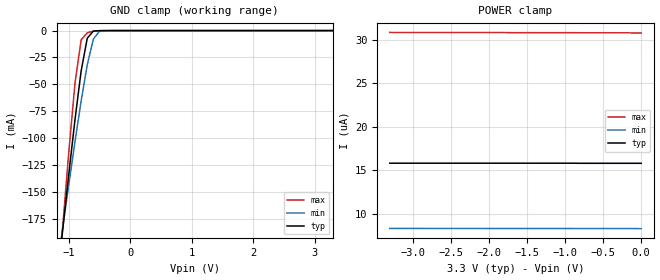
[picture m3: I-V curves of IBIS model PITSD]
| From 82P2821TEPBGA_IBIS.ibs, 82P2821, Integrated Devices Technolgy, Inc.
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|   Model PITSD
[Model]		PITSD
Model_type	Input
Polarity   Non-Inverting
Vinl = 		0.8000V
Vinh = 		2.0000V
C_comp   4.8700pF   4.3000pF   5.3800pF
[Temperature Range]	  25.0000   90.0000   -40.0000
[Voltage Range]   3.3000V   3.0000V   3.6000V
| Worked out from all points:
|   GND clamp passes 1 mA (typ) near -0.61 V on its own axis
[GND_clamp]
|Voltage	  I(typ)   I(min)   I(max)
-3.3V     -1.417A    -1.129A    -1.858A
-1.2V     -239.2mA   -225mA     -255.1mA
-1.1V     -185.7mA   -183.7mA   -182.6mA
-1V       -133.3mA   -143.1mA   -112.7mA
-900mV    -83.07mA   -103.5mA   -49.11mA
-800mV    -37.76mA   -65.72mA   -8.683mA
-700mV    -7.08mA    -31.79mA   -2.043mA
-600mV    -441.5uA   -7.708mA   -455.2uA
-500mV    -36.4uA    -560.8uA   -62.09uA
3.3V      15.8uA     8.301uA    30.77uA
[POWER_clamp]
|Voltage	  I(typ)   I(min)   I(max)
-3.3V     15.81uA    8.312uA    30.84uA
-3.2V     15.81uA    8.312uA    30.83uA
-2.6V     15.81uA    8.309uA    30.83uA
-2.5V     15.81uA    8.309uA    30.82uA
-1.8V     15.81uA    8.307uA    30.82uA
-1.7V     15.81uA    8.306uA    30.81uA
-1V       15.81uA    8.304uA    30.81uA
-900mV    15.81uA    8.303uA    30.81uA
-800mV    15.8uA     8.303uA    30.8uA
-300mV    15.8uA     8.301uA    30.8uA
-100mV    15.8uA     8.3uA      30.78uA
0V        15.8uA     8.287uA    30.78uA
